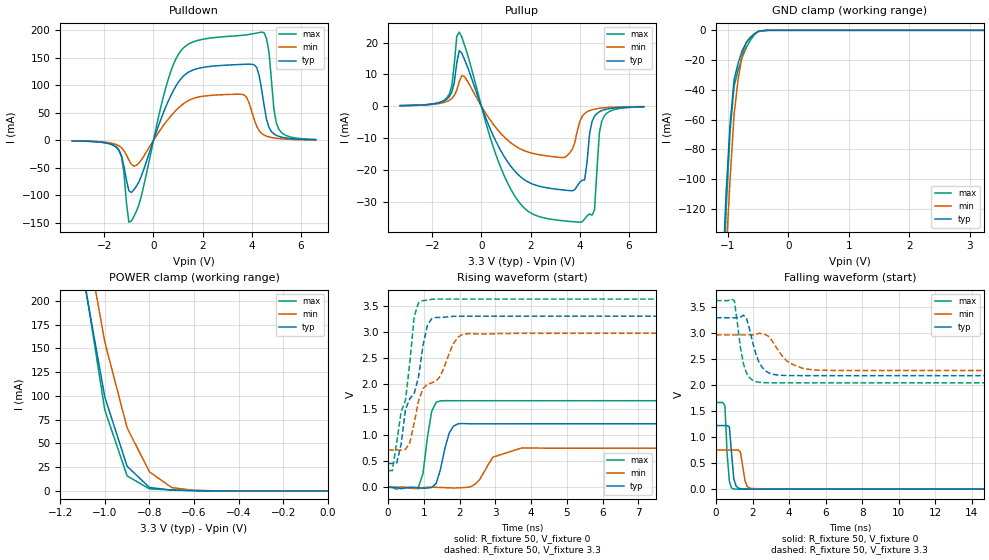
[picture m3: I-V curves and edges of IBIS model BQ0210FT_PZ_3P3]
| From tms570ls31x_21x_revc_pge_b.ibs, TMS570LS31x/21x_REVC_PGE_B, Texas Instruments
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|   Model Cell BQ0210FT_PZ_3P3
|BQ0210FT_PZ_3P3
[Model]   BQ0210FT_PZ_3P3
Model_type   I/O
Polarity   Non-Inverting
Enable   Active-Low
Vinl =  1.15
Vinh =  1.55
Cref =  15.0001pF
Rref =  101.0000M
Vref =  0V
Vmeas =  1.65
C_comp   1.2p   1.2p   1.2p
[Model Spec]
Vinl   1.15   1.02   1.28
Vinh   1.55   1.45   1.65
[Temperature Range]   25   155   -40
[Voltage Range]   3.3   2.97   3.63
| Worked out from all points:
|   slope of the pulldown table from 0 to 0.495 V, typ, clamps not added: 8.21 ohm
|   slope of the pullup table from 0 to 0.495 V, typ, clamps not added: 52.1 ohm
|   GND clamp passes 1 mA (typ) near -0.51 V on its own axis
|   POWER clamp passes 1 mA (typ) near -0.71 V on its own axis
|   rising waveform, R_fixture 50, V_fixture 0: 20-80 % time 261ps typ, 466ps min, 201ps max; typ from 0 V to 1.22 V
|   rising waveform, R_fixture 50, V_fixture 3.3: 20-80 % time 576ps typ, 968ps min, 420ps max; typ from 0.458 V to 3.3 V
|   falling waveform, R_fixture 50, V_fixture 0: 20-80 % time 181ps typ, 214ps min, 167ps max; typ from 1.22 V to 0 V
|   falling waveform, R_fixture 50, V_fixture 3.3: 20-80 % time 29.5ns typ, 31.8ns min, 18.4ns max; typ from 3.3 V to 0.465 V
[POWER_clamp]
|   voltage   I(typ)   I(min)   I(max)
-3.3V     4.048A     4.625A     4.878A
-1.1V     231mA      288.4mA    235.6mA
-1.067V   187mA      244.6mA    185.5mA
-1.033V   143mA      200.7mA    135.4mA
-1V       98.96mA    156.8mA    85.29mA
-900mV    25.97mA    66.53mA    15.83mA
-800mV    3.667mA    20.16mA    2.174mA
-700mV    840.7uA    3.501mA    1.027mA
-600mV    281.5uA    564.5uA    364.3uA
0V        545.1pA    9.477nA    486.7pA
[Pulldown]
|   voltage   I(typ)   I(min)   I(max)
-3.3V     -969uA     -848.2uA   -928.8uA
-1.4V     -17.91mA   -9.953mA   -18.22mA
-1V       -91.46mA   -35.59mA   -148.6mA
-900mV    -94.7mA    -43.39mA   -146.6mA
1.1V      110.9mA    62.3mA     162mA
3.7V      138.3mA    82.11mA    191.3mA
4.2V      132.3mA    25.59mA    195mA
4.4V      92.36mA    12.74mA    196.7mA
4.7V      23.23mA    6.307mA    159.7mA
4.9V      11.73mA    4.459mA    55.98mA
5.1V      7.323mA    3.326mA    20.29mA
6.6V      1.15mA     841.4uA    1.761mA
[Pullup]
|   voltage   I(typ)   I(min)   I(max)
-3.3V     170.4uA    161.9uA    202.8uA
-1.4V     2.221mA    1.492mA    2.652mA
-900mV    17.47mA    7.707mA    23.31mA
500mV     -9.587mA   -5.844mA   -13.22mA
1.4V      -20.78mA   -12.62mA   -28.76mA
3.4V      -26.42mA   -16.07mA   -36.11mA
4V        -23.95mA   -4.814mA   -36.5mA
4.2V      -23.22mA   -2.294mA   -35.5mA
4.6V      -3.167mA   -930.7uA   -32.71mA
4.8V      -1.739mA   -669.4uA   -8.284mA
5V        -1.12mA    -503.2uA   -3.036mA
6.6V      -167.4uA   -126.3uA   -220.9uA
[GND_clamp]
|   voltage   I(typ)   I(min)   I(max)
-3.3V     -3.252A    -2.876A    -4.947A
-1.1V     -174mA     -209.6mA   -199.1mA
-1.033V   -110.1mA   -151.3mA   -121.8mA
-966.7mV  -63.23mA   -100.2mA   -67.91mA
-900mV    -33.37mA   -56.38mA   -37.45mA
-833.3mV  -22.08mA   -33.01mA   -26.8mA
-766.7mV  -13.79mA   -16.89mA   -18.23mA
-700mV    -8.483mA   -8.005mA   -11.74mA
-566.7mV  -2.39mA    -2.398mA   -3.17mA
-500mV    -626.7uA   -905.1uA   -720.5uA
-300mV    -1.304uA   -11.33uA   -645nA
3.233V    524.1pA    1.124uA    388.8pA
[Ramp]
| variable   typ   min   max
dV/dt_f   1.740505/29.50414n   0.5635823/0.4680981n   2.030328/18.34784n
dV/dt_r   0.757382/0.2541379n  0.4745695/0.4317467n   1.026122/0.193933n
R_load = 50
[Rising Waveform]
R_fixture = 50
V_fixture = 0
V_fixture_min = 0
V_fixture_max = 0
|   time   V(typ)   V(min)   V(max)
0s        -18.21uV   -9.233uV   -4.528uV
852ps     -9.378mV   -23.52mV   3.679mV
976ps     -18.75mV   -7.204mV   262.1mV
1.22ns    -3.97mV    1.014mV    1.464V
1.464ns   340.6mV    -4.062mV   1.667V
1.708ns   1.042V     -11.47mV   1.67V
2.076ns   1.229V     -7.496mV   1.669V
2.932ns   1.223V     581.3mV    1.669V
3.744ns   1.224V     758.8mV    1.669V
35.6ns    1.224V     753.2mV    1.669V
[Rising Waveform]
R_fixture = 50
V_fixture = 3.3
V_fixture_min = 2.97
V_fixture_max = 3.63
|   time   V(typ)   V(min)   V(max)
0s        457.6mV    717.1mV    322mV
120ps     457.6mV    717.1mV    321.3mV
244ps     469.7mV    717.1mV    877.6mV
488ps     1.505V     734.2mV    1.682V
732ps     1.813V     1.242V     3.298V
976ps     2.731V     1.904V     3.601V
1.22ns    3.252V     2.014V     3.624V
1.956ns   3.299V     2.895V     3.63V
2.32ns    3.299V     2.964V     3.63V
35.6ns    3.3V       2.97V      3.63V
[Falling Waveform]
R_fixture = 50
V_fixture = 0
V_fixture_min = 0
V_fixture_max = 0
|   time   V(typ)   V(min)   V(max)
0s        1.224V     753.2mV    1.669V
488ps     1.224V     753.2mV    1.607V
608ps     1.223V     753.1mV    693.9mV
732ps     1.201V     753.1mV    152.6mV
976ps     199.8mV    752.5mV    3.317mV
1.1ns     61.15mV    752.8mV    1.234mV
1.344ns   9.094mV    706.3mV    823.4uV
1.588ns   2.205mV    165.1mV    982.7uV
1.956ns   741.7uV    12.27mV    661.2uV
35.6ns    157uV      3.513uV    2.067uV
[Falling Waveform]
R_fixture = 50
V_fixture = 3.3
V_fixture_min = 2.97
V_fixture_max = 3.63
|   time   V(typ)   V(min)   V(max)
0s        3.3V       2.97V      3.63V
1.008ns   3.299V     2.97V      3.628V
1.512ns   3.35V      2.97V      2.4V
2.18ns    2.604V     2.977V     2.071V
18.06ns   2.185V     2.285V     2.051V
20.81ns   2.185V     2.285V     476.9mV
29.14ns   2.188V     2.285V     345mV
34.83ns   551.4mV    2.285V     344.8mV
35.93ns   525.4mV    755.6mV    344.8mV
36.81ns   465.4mV    755.6mV    344.8mV
